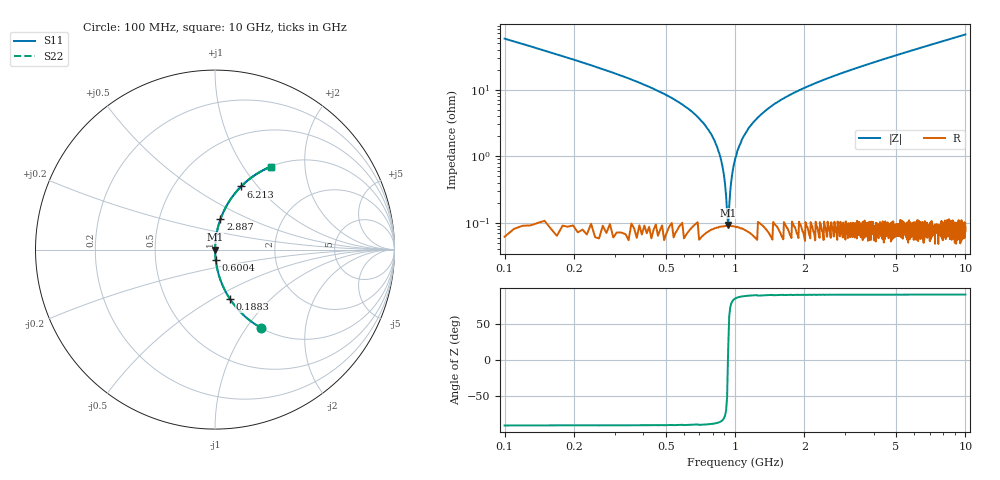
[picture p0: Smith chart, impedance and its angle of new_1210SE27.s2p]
!	AVX	Thin	Film	Operation	Date:	April 2007
!	Description:	Accu-P®	"Series,"	Thin	"Film,"	"SMD,"	RF	Capacitor
!	Part	Number:	12101J270FBT
!	100	MHz	-	5.05	GHz
!	Serial	Measurements
#	MHZ	S	MA	R	50
!	S11	S21	S12	S22
!	dB	Phase	dB	Phase	dB	Phase	dB	Phase
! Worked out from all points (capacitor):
!   1010 points, 100 MHz to 10 GHz, reference 50 ohm
!   read as one part in series: C = 27 pF near 149.1 MHz
!   lowest |Z| = 92.8 mohm at 934 MHz (marker M1)
!   series resonance near 932.3 MHz, so ESL is about 1.1 nH
!   S11 on the Smith chart (normalised r, x): 100 MHz: 1.00, -1.17; 188.3 MHz: 1.00, -0.60; 600.4 MHz: 1.00, -0.11; 2.887 GHz: 1.00, +0.35; 6.213 GHz: 1.00, +0.82; 10 GHz: 1.00, +1.35
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100  0.503 -59.7  0.864 30.2  0.864 30.2  0.503 -59.7
188.305  0.287 -73.1  0.957 16.7  0.957 16.7  0.287 -73.1
345.292  0.146 -81.3  0.989 8.4  0.989 8.4  0.146 -81.3
600.396  0.057 -85.9  0.998 3.3  0.998 3.3  0.057 -85.9
718.137  0.033 -86.7  0.999 1.9  0.999 1.9  0.033 -86.7
806.442  0.018 -86.5  0.999 1.1  0.999 1.1  0.018 -86.5
855.5  0.011 -85.2  0.999 0.6  0.999 0.6  0.011 -85.2
894.747  0.00526 -81.0  0.999 0.3  0.999 0.3  0.00526 -81.0
933.994  0.00083 15.5  0.999 -0.0  0.999 -0.0  0.00083 15.5
963.429  0.00422 78.8  0.999 -0.2  0.999 -0.2  0.00422 78.8
1002.676  0.00923 84.5  0.999 -0.5  0.999 -0.5  0.00923 84.5
1041.923  0.014 85.9  0.999 -0.8  0.999 -0.8  0.014 85.9
1169.475  0.029 86.8  0.999 -1.7  0.999 -1.7  0.029 86.8
1424.579  0.055 86.0  0.998 -3.2  0.998 -3.2  0.055 86.0
1758.176  0.085 84.6  0.996 -4.9  0.996 -4.9  0.085 84.6
2886.521  0.173 79.8  0.984 -9.9  0.984 -9.9  0.173 79.8
3406.541  0.209 77.7  0.977 -12.1  0.977 -12.1  0.209 77.7
5054.906  0.314 71.6  0.949 -18.3  0.949 -18.3  0.314 71.6
6212.686  0.381 67.5  0.924 -22.4  0.924 -22.4  0.381 67.5
6703.271  0.407 65.9  0.913 -24.0  0.913 -24.0  0.407 65.9
8351.635  0.488 60.7  0.872 -29.2  0.872 -29.2  0.488 60.7
10000  0.558 56.0  0.829 -33.9  0.829 -33.9  0.558 56.0
